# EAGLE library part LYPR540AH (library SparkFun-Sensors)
3-axis 400/1600 deg/s analog output gyroscope
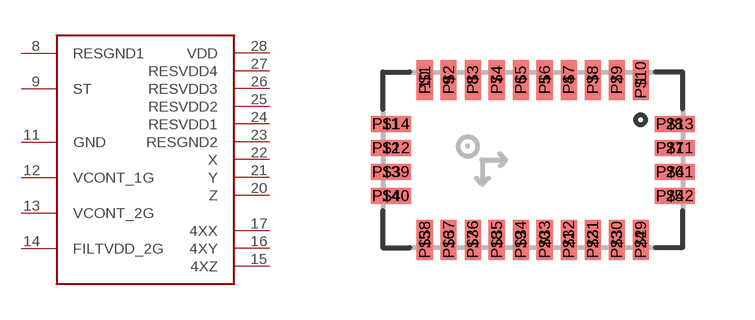
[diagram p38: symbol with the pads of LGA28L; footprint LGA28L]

Designator prefix -

## LYPR540AH  [LGA28L]
8  RESGND1
9  ST
11  GND
12  VCONT_1G
13  VCONT_2G
14  FILTVDD_2G
15  4XZ
16  4XY
17  4XX
20  Z
21  Y
22  X
23  RESGND2
24  RESVDD1
25  RESVDD2
26  RESVDD3
27  RESVDD4
28  VDD

## Footprint LGA28L (pad centres in mm)
smd 0.4 x 1: 1 2.7,2; 2 2.1,2; 3 1.5,2; 4 0.9,2; 5 0.3,2; 6 -0.3,2; 7 -0.9,2; 8 -1.5,2; 9 -2.1,2; 10 -2.7,2; 15 -2.7,-2; 16 -2.1,-2; 17 -1.5,-2; 18 -0.9,-2; 19 -0.3,-2; 20 0.3,-2; 21 0.9,-2; 22 1.5,-2; 23 2.1,-2; 24 2.7,-2; P$1 -2.7,2; P$2 -2.1,2; P$3 -1.5,2; P$4 -0.9,2; P$5 -0.3,2; P$6 0.3,2; P$7 0.9,2; P$8 1.5,2; P$9 2.1,2; P$10 2.7,2; P$29 2.7,-2; P$30 2.1,-2; P$31 1.5,-2; P$32 0.9,-2; P$33 0.3,-2; P$34 -0.3,-2; P$35 -0.9,-2; P$36 -1.5,-2; P$37 -2.1,-2; P$38 -2.7,-2
smd 1 x 0.4: 11 -3.55,0.9; 12 -3.55,0.3; 13 -3.55,-0.3; 14 -3.55,-0.9; 25 3.55,-0.9; 26 3.55,-0.3; 27 3.55,0.3; 28 3.55,0.9; P$11 3.55,0.3; P$12 -3.55,0.3; P$13 3.55,0.9; P$14 -3.55,0.9; P$39 -3.55,-0.3; P$40 -3.55,-0.9; P$41 3.55,-0.3; P$42 3.55,-0.9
